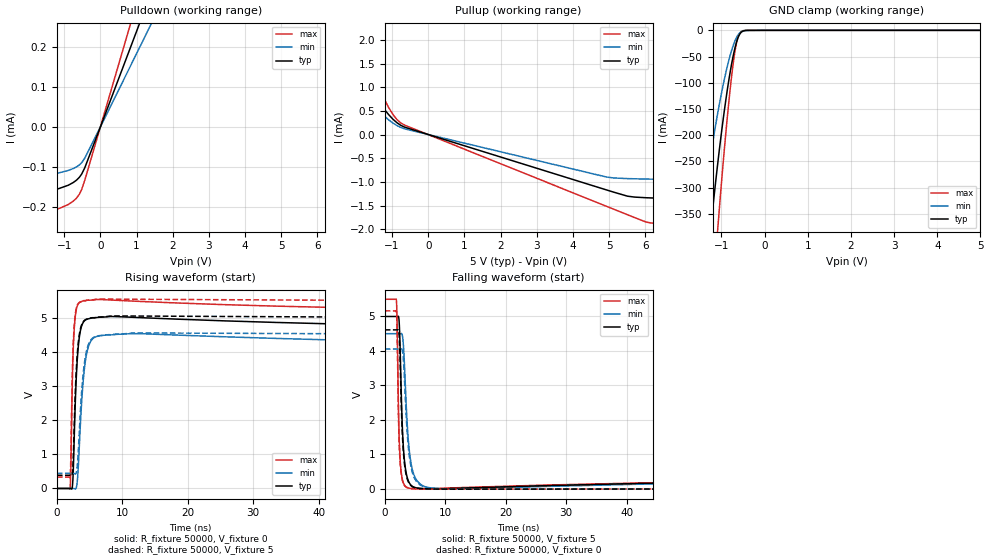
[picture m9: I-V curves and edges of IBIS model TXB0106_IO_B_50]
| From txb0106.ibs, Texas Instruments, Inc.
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[Model]   TXB0106_IO_B_50
Model_type  I/O
Vinl=1.575
Vinh=3.575
Enable   Active-High
Vref =   0
Rref =   1e6
Cref =   15p
Vmeas =   2.5
| variable   typ   min   max
C_comp   13.34pF   11.24pF   15.52pF
| C_pullup   13.27pF   11.21pF   16.01pF
| C_pulldown   23.02pF   10.60pF   39.75pF
| C_tri-state   13.34pF   11.24pF   15.52pF
[Temperature Range]   40   100   -40
| Ambient temperature   25   85   -40
[Voltage range]   5   4.5   5.5
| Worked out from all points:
|   slope of the pulldown table from 0 to 0.75 V, typ, clamps not added: 4.19 kohm
|   slope of the pullup table from 0 to 0.75 V, typ, clamps not added: 4.21 kohm
|   GND clamp passes 1 mA (typ) near -0.48 V on its own axis
|   rising waveform, R_fixture 50000, V_fixture 0: 20-80 % time 520ps typ, 750ps min, 335ps max; typ from 0 V to 4.62 V
|   falling waveform, R_fixture 50000, V_fixture 5: 20-80 % time 504ps typ, 751ps min, 324ps max; typ from 5 V to 0.374 V
|   rising waveform, R_fixture 50000, V_fixture 5: 20-80 % time 606ps typ, 901ps min, 380ps max; typ from 0.386 V to 5 V
|   falling waveform, R_fixture 50000, V_fixture 0: 20-80 % time 602ps typ, 934ps min, 371ps max; typ from 4.61 V to -0.001 V
[GND Clamp]
| TXB0104_IO_B_50
|   Voltage   I(typ)   I(min)   I(max)
-5.5V     -5.138A    -3.901A    -6.439A
-1.49V    -586.5mA   -378.2mA   -853.1mA
-1.46V    -559.5mA   -359.9mA   -815.8mA
-1.235V   -368.5mA   -232.3mA   -546.8mA
-1.095V   -262.3mA   -163.1mA   -391.6mA
-1.07V    -244.6mA   -151.7mA   -365.3mA
-890mV    -129.5mA   -78.65mA   -190.6mA
-735mV    -52.65mA   -31.4mA    -69.36mA
-675mV    -30.55mA   -18.44mA   -35.49mA
-625mV    -16.62mA   -10.47mA   -16.26mA
-520mV    -2.469mA   -1.958mA   -1.335mA
5V        1.546nA    6.018nA    161.4pA
[Pulldown]
| TXB0104_IO_B_50
|   Voltage   I(typ)   I(min)   I(max)
-5.5V     -217uA     -165uA     -283uA
-4.41V    -206uA     -156uA     -268uA
-3.195V   -190uA     -144uA     -251uA
-2.12V    -174uA     -130.6uA   -231uA
-1.275V   -157.6uA   -117.3uA   -208.6uA
-885mV    -145.1uA   -108.1uA   -193.2uA
-660mV    -132.6uA   -99.43uA   -177.5uA
-580mV    -125.4uA   -94.46uA   -167.8uA
-515mV    -117.2uA   -88.7uA    -155.6uA
-430mV    -101.7uA   -77.55uA   -132.8uA
0V        0A         0A         0A
11V       2.628mA    2.017mA    3.403mA
[Pullup]
| TXB0104_IO_B_50
|   Voltage   I(typ)   I(min)   I(max)
-5.5V     11.53mA    5.155mA    20.58mA
-2.415V   3.372mA    2.27mA     4.905mA
-2.165V   2.318mA    1.621mA    3.274mA
-1.925V   1.595mA    1.145mA    2.308mA
-1.68V    1.13mA     810uA      1.669mA
-1.205V   528.2uA    386.5uA    736.9uA
-865mV    252.4uA    192.7uA    319.7uA
-645mV    156.2uA    120.9uA    199.2uA
4.92V     -1.165mA   -893.5uA   -1.511mA
5.51V     -1.3mA     -927.9uA   -1.692mA
6.025V    -1.332mA   -937.3uA   -1.845mA
11V       -1.392mA   -979uA     -1.958mA
[Ramp]
| TXB0104_IO_B_50
| variable   typ   min   max
dV/dt_r   3.04/6.33E-10   2.73/9.41E-10   3.34/3.99E-10
dV/dt_f   3.01/6.13E-10   2.70/9.51E-10   3.31/3.79E-10
R_load = 50000
[Rising Waveform]
| TXB0104_IO_B_50
R_fixture =   50000
C_fixture =   0
L_fixture =   0
V_fixture =   0
V_fixture_min = 0
V_fixture_max = 0
|   Time   V(typ)   V(min)   V(max)
0s        221.3nV    1.663uV    67.5nV
2.02ns    302.2uV    23.12uV    18.34mV
2.125ns   -737.8uV   50.32uV    547.6mV
2.485ns   437.8mV    1.057mV    4.018V
2.99ns    3.357V     43.68mV    5.269V
3.565ns   4.599V     1.788V     5.465V
4.04ns    4.876V     3.197V     5.503V
4.595ns   4.963V     3.999V     5.519V
11.74ns   5.019V     4.543V     5.494V
220ns     4.616V     4.071V     5.165V
[Falling Waveform]
| TXB0104_IO_B_50
R_fixture =   50000
C_fixture =   0
L_fixture =   0
V_fixture =   5
V_fixture_min = 4.5
V_fixture_max = 5.5
|   Time   V(typ)   V(min)   V(max)
0s        5V         4.5V       5.5V
1.915ns   5V         4.5V       5.476V
2.04ns    4.999V     4.5V       4.799V
2.305ns   4.973V     4.5V       1.956V
2.595ns   3.672V     4.499V     697.7mV
3.115ns   1.097V     4.062V     150.4mV
3.77ns    289.1mV    1.698V     30.62mV
4.365ns   96.86mV    714.2mV    5.944mV
10.96ns   6.74mV     -2.249mV   22.26mV
220ns     373.6mV    411.4mV    329.7mV
[Rising Waveform]
| TXB0104_IO_B_50
R_fixture =   50000
C_fixture =   0
L_fixture =   0
V_fixture =   5
V_fixture_min = 4.5
V_fixture_max = 5.5
|   Time   V(typ)   V(min)   V(max)
0s        386.1mV    442.3mV    333.9mV
2.01ns    386.4mV    442.3mV    333.8mV
2.125ns   385.4mV    442.4mV    885.4mV
2.33ns    399.3mV    442.4mV    3.119V
2.66ns    1.943V     438.2mV    4.808V
3.215ns   4.175V     918.6mV    5.411V
3.865ns   4.838V     3.046V     5.496V
4.555ns   4.967V     4.056V     5.521V
12.36ns   5.056V     4.561V     5.548V
220ns     5.001V     4.502V     5.5V
[Falling Waveform]
| TXB0104_IO_B_50
R_fixture =   50000
C_fixture =   0
L_fixture =   0
V_fixture =   0
V_fixture_min = 0
V_fixture_max = 0
|   Time   V(typ)   V(min)   V(max)
0s        4.611V     4.054V     5.164V
1.915ns   4.611V     4.054V     5.141V
2.305ns   4.585V     4.054V     1.758V
2.59ns    3.338V     4.054V     638.6mV
3.1ns     1.005V     3.665V     141.3mV
3.73ns    272.1mV    1.559V     29.3mV
4.33ns    88.42mV    642.4mV    4.193mV
6.205ns   1.028mV    72.69mV    -8.549mV
12.39ns   -13.1mV    -13.29mV   -10.85mV
220ns     -517.5uV   -1.214mV   -179.8uV
